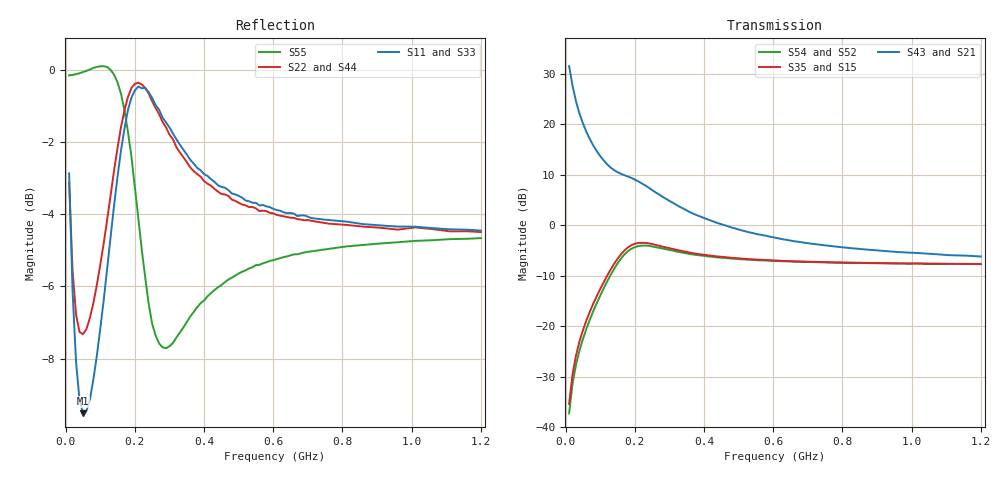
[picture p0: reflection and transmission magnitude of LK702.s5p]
! Date: Wed May 20 11:25:11 1998
!  POLYFET RF DEVICES
!  LP702/LK702
!  28Vdc		400ma
!AWR Design Environment (2053) Wed Feb 04 14:51:57 2004
!freq-unit  param-type  data-format  keyword  impedance-ohms
# MHz  S  MA  R  50
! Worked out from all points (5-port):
!   120 points, 10 MHz to 1.2 GHz, reference 50 ohm
!   strongest paths, dB at 10 MHz, 310 MHz, 610 MHz, 910 MHz, 1.2 GHz:
!     S43: 31.5, 4.4, -2.6, -5.1, -6.2
!     S21: 31.5, 4.4, -2.6, -5.1, -6.2
!     S35: -35.4, -4.7, -7.0, -7.5, -7.7
!     S15: -35.4, -4.7, -7.0, -7.5, -7.7
!     S54: -37.3, -5.1, -7.1, -7.6, -7.7
!     S52: -37.3, -5.1, -7.1, -7.6, -7.7
!   lowest |S11| = -9.5 dB at 50 MHz (marker M1), VSWR 2.01, Z = 55.2 - j36.9 ohm
!   |S11| at or under -10 dB: nowhere
